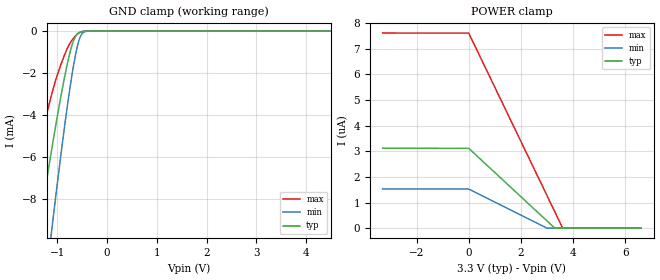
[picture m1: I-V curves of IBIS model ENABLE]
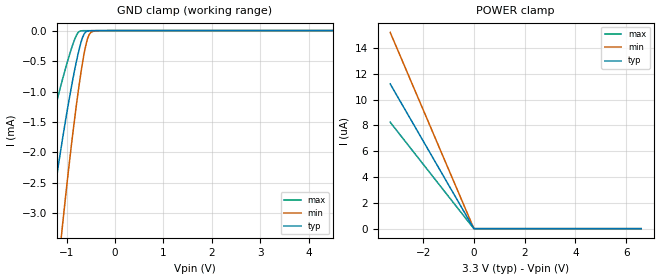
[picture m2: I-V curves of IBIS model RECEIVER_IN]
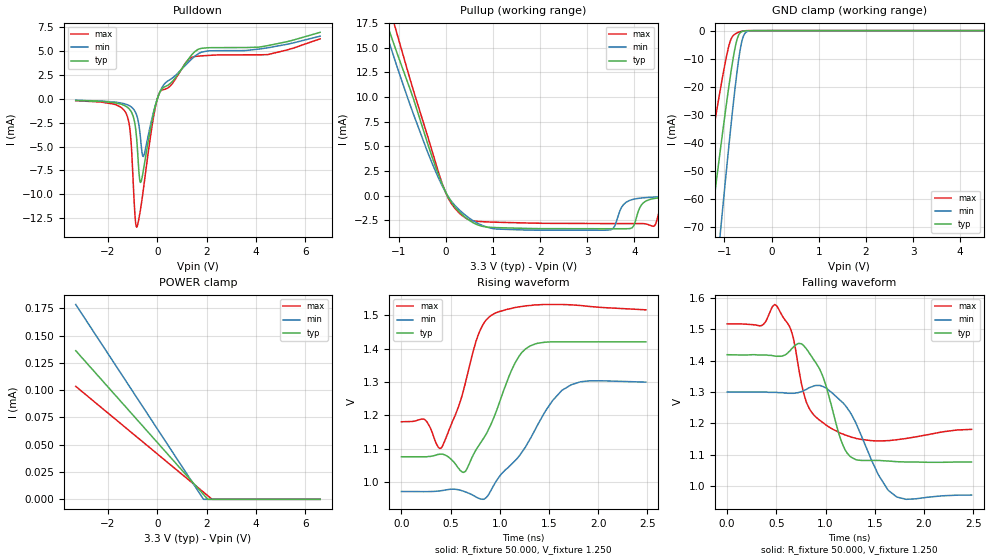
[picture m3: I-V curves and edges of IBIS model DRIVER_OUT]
|Texas Instruments Incorporated
|IBIS model for SN65LVDS104
|4-PORT LVDS and 4-PORT TTL-TO-LVDS REPEATERS
| Marketing part#   Voltage Range   Package-type   #pins/pkg drawing
| SN65LVDS104D   3.0V - 3.6V   SOIC   16-pin
| SN65LVDS104DG4   3.0V - 3.6V   SOIC   16-pin
| SN65LVDS104DR   3.0V - 3.6V   SOIC   16-pin
| SN65LVDS104DRG4   3.0V - 3.6V   SOIC   16-pin
| SN65LVDS104PW   3.0V - 3.6V   TSSOP   16-pin
| SN65LVDS104PWG4   3.0V - 3.6V   TSSOP   16-pin
| SN65LVDS104PWR   3.0V - 3.6V   TSSOP   16-pin
| SN65LVDS104PWRG4   3.0V - 3.6V   TSSOP   16-pin
[IBIS Ver]   4.0
[File name]   sn65lvds104.ibs
[File Rev]   3.1
[Date]   03/25/2009
[Source]   Texas Instruments Incorporated.
   Analog-eLab, HPA
   12500 TI Blvd
   Dallas, TX -75243
   For Support e-mail: elab_ibis@list.ti.com
[Notes]   Revision History:
   05/09/2006: Rev 3.0 to correct errors
   - Old revision on the web until March 2009
   - Created by Data transmissions Group
   03/25/2009: Rev 3.1
   - Updated model with corner buffer models
   - removed capactive load while generating V-T waveforms
   for DRIVER_OUT model
   - All buffer models updated with ccomp and new buffer data
   - Header, Source, Notes, Disclaimer updated
   - New package models for SOIC and TSSOP packages
   - TSSOP models added to IBIS file
   - ccomp min and max values are based on PVT conditions and are
   as per simulations in TISPICE
   - Models are based on simulations in TISPICE
   - Models not matched to measurements
   - Models revisioned back to 1.1, since it is not matched to measurements
   - Warnings related to no-monotonicity reflect true buffer
   behavior
   - Added Undershoot and Overshoot parameters, for DRIVER_OUT they
   are commented out
[Disclaimer] This model is designed as an aid for customers of Texas Instruments.
 TI and its licensors and suppliers make no warranties, either expressed
 or implied, with respect to this  model, including the warranties of
 merchantability or fitness for a particular purpose.
 The model is provided solely on an "as is" basis. The entire risk as to
 its quality and performance is with the customer.
[Copyright] (C)Copyright 2009 Texas Instruments Incorporated. All rights reserved.
|   SN65LVDS104D Component
[Component]   SN65LVDS104D
[Manufacturer]  Texas Instruments Incorporated
[Package]   |16-pin SOIC - 'D' package
|   typ   min   max
R_pkg   0.1501   0.12041   0.17979
L_pkg   2.815455nH   1.96433nH   3.66658nH
C_pkg   0.4138pF   0.24048pF   0.58712nH
[Pin]   signal_name   model_name   R_pin   L_pin   C_pin
   1   EN1   ENABLE   0.17868  3.66658nH  0.58598pF
   2   EN2   ENABLE   0.17508  3.07679nH  0.42614pF
   3   EN3   ENABLE   0.16515  2.40747nH  0.25884pF
   4   VCC   POWER   0.06487  1.66922nH  0.27036pF
   5   GND   GND   0.06582  1.67357nH  0.27362pF
   6   A   RECEIVER_IN   0.16724  2.43491nH  0.26090pF
   7   B   RECEIVER_IN   0.17430  3.07526nH  0.42629pF
   8   EN4   ENABLE   0.17833  3.66652nH  0.58506pF
   9   4Z   DRIVER_OUT   0.17601  3.64076nH  0.58692pF
   10   4Y   DRIVER_OUT   0.17979  3.12894nH  0.43064pF
   11   3Z   DRIVER_OUT   0.17292  2.49311nH  0.26155pF
   12   3Y   DRIVER_OUT   0.12171  1.97811nH  0.24138pF
   13   2Z   DRIVER_OUT   0.12041  1.96433nH  0.24048pF
   14   2Y   DRIVER_OUT   0.16249  2.38061nH  0.25661pF
   15   1Z   DRIVER_OUT   0.17971  3.12362nH  0.42991pF
   16   1Y   DRIVER_OUT   0.17545  3.63250nH  0.58712pF
|   SN65LVDS104PW Component
[Component]   SN65LVDS104PW
[Manufacturer]  Texas Instruments Incorporated
[Package]   |16-pin TSSOP - 'PW' package
|   typ   min   max
R_pkg   0.170335   0.1467   0.19397
L_pkg   2.751175nH   2.29411nH   3.20824nH
C_pkg   0.477225pF   0.44752pF   0.50693pF
[Pin]   signal_name   model_name   R_pin   L_pin   C_pin
   1   EN1   ENABLE   0.17988  3.18805nH  0.50544pF
   2   EN2   ENABLE   0.16953  2.53112nH  0.44901pF
   3   EN3   ENABLE   0.15255  2.35283nH  0.45699pF
   4   VCC   POWER   0.07840  1.93255nH  0.48253pF
   5   GND   GND   0.08071  1.96120nH  0.48761pF
   6   A   RECEIVER_IN   0.15344  2.36420nH  0.45832pF
   7   B   RECEIVER_IN   0.16626  2.50189nH  0.44752pF
   8   EN4   ENABLE   0.17863  3.18204nH  0.50510pF
   9   4Z   DRIVER_OUT   0.18112  3.20824nH  0.50693pF
   10   4Y   DRIVER_OUT   0.19397  2.78352nH  0.46026pF
   11   3Z   DRIVER_OUT   0.15624  2.39243nH  0.45899pF
   12   3Y   DRIVER_OUT   0.14670  2.29411nH  0.45418pF
   13   2Z   DRIVER_OUT   0.14708  2.29825nH  0.45398pF
   14   2Y   DRIVER_OUT   0.15170  2.34450nH  0.45668pF
   15   1Z   DRIVER_OUT   0.19359  2.77669nH  0.46057pF
   16   1Y   DRIVER_OUT   0.17990  3.18836nH  0.50665pF
[Diff_pin]   inv_pin   vdiff   tdelay_typ   tdelay_min   tdelay_max
| The 'xA' or 'xY' pins are Diff_pins and the 'xB' or 'xZ' pins are inv_pins
6   7   0.100   0 0 0
10   9   0.100   0 0 0
12   11   0.100   0 0 0
14   13   0.100   0 0 0
16   15   0.100   0 0 0
| Models and submodels in the file (3): ENABLE (Input), RECEIVER_IN (Input), DRIVER_OUT (3-state)
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|   Driver Enable MODEL
[Model]   ENABLE
Model_type   Input
|Signals   EN1,EN2,EN3,EN4
Vinh = 2.0
Vinl = 0.8
|   typ   min   max
C_comp   0.6100pF   0.6494pF   0.5720pF
[Model spec]
|Overshoot
S_overshoot_high   6V   6V   6V
S_overshoot_low   -0.5V   -0.5V   -0.5V
|   typ   min   max
|Ambient temperature   25C   85C   -40C
[Temperature Range]   40   100   -40
[Voltage range]   3.3V   3.0V   3.6V
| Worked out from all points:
|   GND clamp passes 1 mA (typ) near -0.74 V on its own axis
[GND Clamp]
|   Voltage   I(typ)   I(min)   I(max)
-3.3V     -44.67mA   -64.4mA    -29.86mA
-1.795V   -16.37mA   -24.59mA   -10.37mA
-1.691V   -14.64mA   -22.16mA   -9.17mA
-1.365V   -9.426mA   -14.83mA   -5.55mA
-1.107V   -5.596mA   -9.439mA   -2.987mA
-929mV    -3.158mA   -5.962mA   -1.619mA
-760.7mV  -1.189mA   -2.989mA   -652.8uA
-656.7mV  -365.7uA   -1.444mA   -299uA
-542.9mV  -46.55uA   -316.6uA   -65.84uA
-478.5mV  -12.23uA   -73.15uA   -17.6uA
-354.8mV  -1.564uA   -2.63uA    -2.722uA
6.595V    0A         0A         0A
[POWER Clamp]
|   Voltage   I(typ)   I(min)   I(max)
-3.3V     3.125uA    1.534uA    7.623uA
0V        3.117uA    1.526uA    7.616uA
3.001V    280.8nA    0A         1.267uA
3.298V    0A         0A         639nA
3.6V      0A         0A         0A
6.595V    0A         0A         0A
|   Receiver Input MODEL
[Model]   RECEIVER_IN
Model_type   Input
|Signals   A,B
Vinh = 1.3
Vinl = 1.1
|   typ   min   max
C_comp   1.1515pF   1.2187pF   1.1001pF
[Model spec]
|Overshoot
S_overshoot_high   4V   4V   4V
S_overshoot_low   -0.5V   -0.5V   -0.5V
|   typ   min   max
|Ambient temperature   25C   85C   -40C
[Temperature Range]   40   100   -40
[Voltage range]   3.3V   3.0V   3.6V
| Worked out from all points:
|   GND clamp passes 1 mA (typ) near -0.92 V on its own axis
[GND Clamp]
|   Voltage   I(typ)   I(min)   I(max)
-3.3V     -19.34mA   -29.51mA   -11.41mA
-1.795V   -6.034mA   -9.654mA   -3.358mA
-1.766V   -5.829mA   -9.345mA   -3.234mA
-1.389V   -3.432mA   -5.716mA   -1.792mA
-1.35V    -3.202mA   -5.367mA   -1.654mA
-1.092V   -1.819mA   -3.257mA   -823.7uA
-854.7mV  -732.7uA   -1.579mA   -190.6uA
-716.1mV  -232.3uA   -757uA     -6.664uA
-636.9mV  -55.35uA   -373.5uA   -1.685uA
-567.6mV  -8.004uA   -134.6uA   -1.413uA
-399.3mV  -1.365uA   -3.155uA   -992nA
6.595V    0A         0A         0A
[POWER Clamp]
|   Voltage   I(typ)   I(min)   I(max)
-3.3V     11.21uA    15.2uA     8.249uA
-3.285V   11.14uA    15.11uA    8.199uA
0V        0A         0A         0A
6.595V    0A         0A         0A
|   Driver Output  MODEL
[Model]   DRIVER_OUT
Model_type   3-state
| Signals   1Y,1Z,2Y,2Z,3Y,3Z,4Y,4Z
Vmeas = 1.2V   |Reference voltage for timing measurements
Cref = 10pF   |Timing specification test load capacitance value
Rref = 50   |Note: 50 Ohm load; single ended configuration
Vref = 1.225V   |Timing specification test load voltage
| variable   typ   min   max
|Driver Enabled
C_comp   4.008pF   3.9392pF   4.1419pF
|Driver Disabled
|C_comp   2.5847pF   2.6537pF   2.5288pF
|[Model spec]
||Overshoot
|S_overshoot_high   4V   4V   4V
|S_overshoot_low   -0.5V   -0.5V   -0.5V
|   typ   min   max
|Ambient temperature   25C   85C   -40C
[Temperature Range]   40   100   -40
[Voltage range]   3.3V   3.0V   3.6V
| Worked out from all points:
|   slope of the pulldown table from 0 to 0.495 V, typ, clamps not added: 316 ohm
|   slope of the pullup table from 0 to 0.495 V, typ, clamps not added: 175 ohm
|   GND clamp passes 1 mA (typ) near -0.67 V on its own axis
|   falling waveform, R_fixture 50.000, V_fixture 1.250: 20-80 % time 187ps typ, 284ps min, 147ps max; typ from 1.42 V to 1.08 V
|   rising waveform, R_fixture 50.000, V_fixture 1.250: 20-80 % time 283ps typ, 453ps min, 187ps max; typ from 1.08 V to 1.42 V
[Pulldown]
|   Voltage   I(typ)   I(min)   I(max)
-3.3V     -151.5uA   -137uA     -182.8uA
-1.261V   -775.5uA   -559.8uA   -1.511mA
-1.082V   -1.215mA   -782.2uA   -3.774mA
-904.2mV  -2.603mA   -1.285mA   -12.09mA
-829.9mV  -4.286mA   -1.727mA   -13.45mA
-716.1mV  -8.355mA   -3.223mA   -12.18mA
-646.8mV  -8.618mA   -4.934mA   -11.07mA
-537.9mV  -7.118mA   -5.914mA   -9.018mA
0V        -4.257uA   -6.043uA   -2.635uA
1.284V    4.256mA    3.911mA    4.188mA
4.476V    5.595mA    5.366mA    4.654mA
6.595V    6.992mA    6.59mA     6.31mA
[GND Clamp]
|   Voltage   I(typ)   I(min)   I(max)
-3.3V     -355.9mA   -493.8mA   -256.4mA
-1.567V   -107.6mA   -159.5mA   -69.86mA
-1.305V   -71.66mA   -111.3mA   -42.78mA
-1.077V   -41.45mA   -70.6mA    -20.18mA
-958.7mV  -26.4mA    -50.11mA   -9.483mA
-879.4mV  -16.97mA   -36.95mA   -3.99mA
-775.5mV  -6.348mA   -20.81mA   -1.282mA
-706.2mV  -1.961mA   -11.44mA   -644uA
-646.8mV  -564.8uA   -5.216mA   -311.4uA
-602.2mV  -230.8uA   -2.283mA   -160uA
-458.7mV  -48.11uA   -108.4uA   -36.76uA
6.595V    0A         0A         0A
[Pullup]
|   Voltage   I(typ)   I(min)   I(max)
-3.3V     50.08mA    48.33mA    58.58mA
-1.285V   17.93mA    16.81mA    20.73mA
-1.048V   14.63mA    13.26mA    16.62mA
0V        320.4uA    298.9uA    250.3uA
303.6mV   -1.738mA   -1.537mA   -1.859mA
674.8mV   -2.979mA   -2.814mA   -2.619mA
3.501V    -3.368mA   -3.476mA   -2.842mA
3.907V    -3.348mA   -480.4uA   -2.843mA
4.145V    -976.6uA   -252.1uA   -2.844mA
4.397V    -321.1uA   -164.3uA   -3.126mA
4.749V    -157.3uA   -109.2uA   -360uA
6.595V    -39.37uA   -36.95uA   -38.93uA
[POWER Clamp]
|   Voltage   I(typ)   I(min)   I(max)
-3.3V     136.2uA    178.4uA    103.5uA
1.873V    4.475uA    42.81nA    6.564uA
2.051V    0A         0A         3.225uA
2.224V    0A         0A         0A
6.595V    0A         0A         0A
[Ramp]
R_load = 50.00Ohm
|   typ   min   max
dV/dt_r   206.942mV/283.916ps 197.045mV/453.868ps 198.756mV/187.252ps
dV/dt_f   199.246mV/187.036ps 197.045mV/285.370ps 175.529mV/147.139ps
[Falling Waveform]
R_fixture = 50.000
V_fixture = 1.250
V_fixture_min = 1.125
V_fixture_max = 1.375
|  time   V(typ)   V(min)   V(max)
0s        1.419V     1.3V       1.517V
350.9ps   1.418V     1.3V       1.512V
502.5ps   1.414V     1.299V     1.575V
649.6ps   1.436V     1.296V     1.497V
760.2ps   1.453V     1.302V     1.319V
969.4ps   1.352V     1.318V     1.203V
1.157ns   1.146V     1.271V     1.168V
1.311ns   1.084V     1.199V     1.152V
1.724ns   1.078V     965.3mV    1.148V
2.483ns   1.077V     971.7mV    1.181V
[Rising Waveform]
R_fixture = 50.000
V_fixture = 1.250
V_fixture_min = 1.125
V_fixture_max = 1.375
|  time   V(typ)   V(min)   V(max)
0s        1.076V     971.7mV    1.181V
239ps     1.076V     971.4mV    1.187V
403.3ps   1.084V     974.1mV    1.102V
649.6ps   1.032V     970.5mV    1.298V
795.5ps   1.114V     950.1mV    1.453V
950ps     1.202V     996.7mV    1.507V
1.157ns   1.359V     1.065V     1.524V
1.304ns   1.408V     1.128V     1.53V
1.724ns   1.421V     1.292V     1.532V
2.483ns   1.421V     1.3V       1.517V
